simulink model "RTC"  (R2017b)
settings: Solver=FixedStepDiscrete  StartTime=0.0  StopTime=10.0  FixedStep=0.01  RelTol=1e-3  EnableMultiTasking=on
undefined symbols (not defined in the file): ASWTYPE_FALSE, ASWTYPE_TRUE, Enum_CTCCtrCtlState, Enum_ISPEcuOffTiSt, RTC_CONST0_NUMB, RTC_CONST1000_NUMB, RTC_CONST4294967000_NUMB, RTC_CONST60_NUMB, RTC_CONST86400_NUMB, RTC_RUNTIME_MS
libraries: AIWAYS_Powertrain_BMS_lib x32

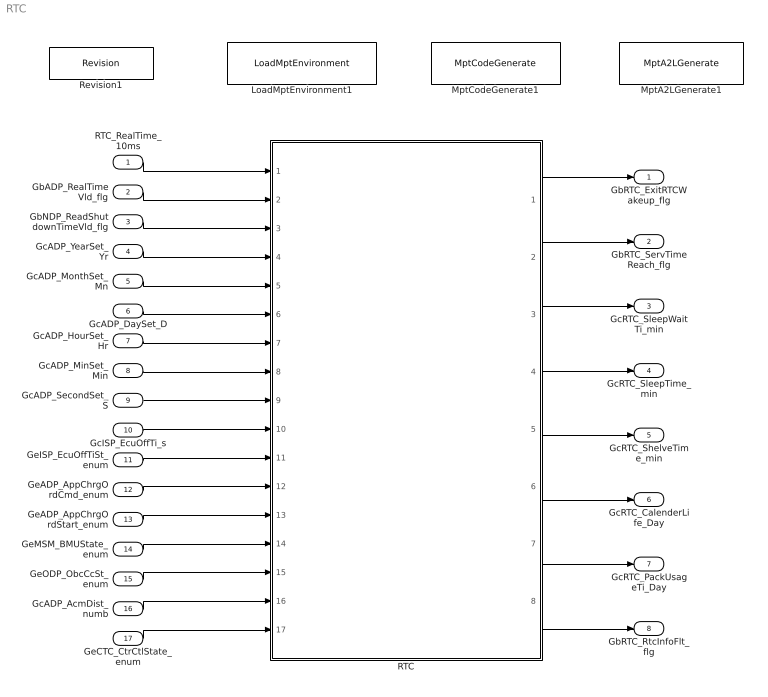
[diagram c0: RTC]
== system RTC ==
  RTC_RealTime_10ms : Inport
  GbADP_RealTimeVld_flg : Inport  Port=2
  GbNDP_ReadShutdownTimeVld_flg : Inport  Port=3
  GcADP_YearSet_Yr : Inport  Port=4
  GcADP_MonthSet_Mn : Inport  Port=5
  GcADP_DaySet_D : Inport  Port=6
  GcADP_HourSet_Hr : Inport  Port=7
  GcADP_MinSet_Min : Inport  Port=8
  GcADP_SecondSet_S : Inport  Port=9
  GcISP_EcuOffTi_s : Inport  Port=10
  GeISP_EcuOffTiSt_enum : Inport  Port=11
  GeADP_AppChrgOrdCmd_enum : Inport  Port=12
  GeADP_AppChrgOrdStart_enum : Inport  Port=13
  GeMSM_BMUState_enum : Inport  Port=14
  GeODP_ObcCcSt_enum : Inport  Port=15
  GcADP_AcmDist_numb : Inport  Port=16
  GeCTC_CtrCtlState_enum : Inport  Port=17
  LoadMptEnvironment1 : AIWAYS_Powertrain_BMS_lib/Config/LoadMptEnvironment  ProjectName=Comm  SuppierID=NewPlatformUAES
  MptA2LGenerate1 : AIWAYS_Powertrain_BMS_lib/Config/MptA2LGenerate  SystemSampleTime=-1
  MptCodeGenerate1 : AIWAYS_Powertrain_BMS_lib/Config/MptCodeGenerate  SystemSampleTime=-1
  RTC : Subsystem
  Revision1 : AIWAYS_Powertrain_BMS_lib/Config/Revision  curVersion='M102C100'  newVersion='M102C100'
  GbRTC_ExitRTCWakeup_flg : Outport
  GbRTC_ServTimeReach_flg : Outport  Port=2
  GcRTC_SleepWaitTi_min : Outport  Port=3
  GcRTC_SleepTime_min : Outport  Port=4
  GcRTC_ShelveTime_min : Outport  Port=5
  GcRTC_CalenderLife_Day : Outport  Port=6
  GcRTC_PackUsageTi_Day : Outport  Port=7
  GbRTC_RtcInfoFlt_flg : Outport  Port=8
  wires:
  RTC_RealTime_10ms/1 -> RTC/1(RTC_RealTime_10ms)
  GbADP_RealTimeVld_flg/1 -> RTC/2(GbADP_RealTimeVld_flg)
  GbNDP_ReadShutdownTimeVld_flg/1 -> RTC/3(GbNDP_ReadShutdownTimeVld_flg)
  GcADP_YearSet_Yr/1 -> RTC/4(GcADP_YearSet_Yr)
  GcADP_MonthSet_Mn/1 -> RTC/5(GcADP_MonthSet_Mn)
  GcADP_DaySet_D/1 -> RTC/6(GcADP_DaySet_D)
  GcADP_HourSet_Hr/1 -> RTC/7(GcADP_HourSet_Hr)
  GcADP_MinSet_Min/1 -> RTC/8(GcADP_MinSet_Min)
  GcADP_SecondSet_S/1 -> RTC/9(GcADP_SecondSet_S)
  GcISP_EcuOffTi_s/1 -> RTC/10(GcISP_EcuOffTi_s)
  GeISP_EcuOffTiSt_enum/1 -> RTC/11(GeISP_EcuOffTiSt_enum)
  GeADP_AppChrgOrdCmd_enum/1 -> RTC/12(GeADP_AppChrgOrdCmd_enum)
  GeADP_AppChrgOrdStart_enum/1 -> RTC/13(GeADP_AppChrgOrdStart_enum)
  GeMSM_BMUState_enum/1 -> RTC/14(GeMSM_BMUState_enum)
  GeODP_ObcCcSt_enum/1 -> RTC/15(GeODP_ObcCcSt_enum)
  GcADP_AcmDist_numb/1 -> RTC/16(GcADP_AcmDist_numb)
  GeCTC_CtrCtlState_enum/1 -> RTC/17(GeCTC_CtrCtlState_enum)
  RTC/1(GbRTC_ExitRTCWakeup_flg) -> GbRTC_ExitRTCWakeup_flg/1
  RTC/2(GbRTC_ServTimeReach_flg) -> GbRTC_ServTimeReach_flg/1
  RTC/3(GcRTC_SleepWaitTi_min) -> GcRTC_SleepWaitTi_min/1
  RTC/4(GcRTC_SleepTime_min) -> GcRTC_SleepTime_min/1
  RTC/5(GcRTC_ShelveTime_min) -> GcRTC_ShelveTime_min/1
  RTC/6(GcRTC_CalenderLife_Day) -> GcRTC_CalenderLife_Day/1
  RTC/7(GcRTC_PackUsageTi_Day) -> GcRTC_PackUsageTi_Day/1
  RTC/8(GbRTC_RtcInfoFlt_flg) -> GbRTC_RtcInfoFlt_flg/1

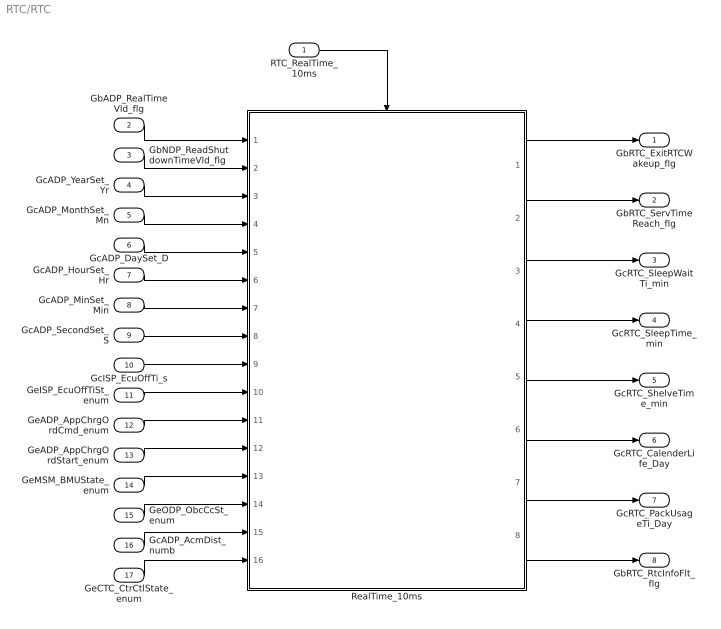
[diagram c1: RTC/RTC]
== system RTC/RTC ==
  RTC_RealTime_10ms : Inport
  GbADP_RealTimeVld_flg : Inport  Port=2
  GbNDP_ReadShutdownTimeVld_flg : Inport  Port=3
  GcADP_YearSet_Yr : Inport  Port=4
  GcADP_MonthSet_Mn : Inport  Port=5
  GcADP_DaySet_D : Inport  Port=6
  GcADP_HourSet_Hr : Inport  Port=7
  GcADP_MinSet_Min : Inport  Port=8
  GcADP_SecondSet_S : Inport  Port=9
  GcISP_EcuOffTi_s : Inport  Port=10
  GeISP_EcuOffTiSt_enum : Inport  Port=11
  GeADP_AppChrgOrdCmd_enum : Inport  Port=12
  GeADP_AppChrgOrdStart_enum : Inport  Port=13
  GeMSM_BMUState_enum : Inport  Port=14
  GeODP_ObcCcSt_enum : Inport  Port=15
  GcADP_AcmDist_numb : Inport  Port=16
  GeCTC_CtrCtlState_enum : Inport  Port=17
  RealTime_10ms : Subsystem
  GbRTC_ExitRTCWakeup_flg : Outport
  GbRTC_ServTimeReach_flg : Outport  Port=2
  GcRTC_SleepWaitTi_min : Outport  Port=3
  GcRTC_SleepTime_min : Outport  Port=4
  GcRTC_ShelveTime_min : Outport  Port=5
  GcRTC_CalenderLife_Day : Outport  Port=6
  GcRTC_PackUsageTi_Day : Outport  Port=7
  GbRTC_RtcInfoFlt_flg : Outport  Port=8
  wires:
  RTC_RealTime_10ms/1 -> RealTime_10ms/Trigger
  GbADP_RealTimeVld_flg/1 -> RealTime_10ms/1(GbADP_RealTimeVld_flg)
  GbNDP_ReadShutdownTimeVld_flg/1 -> RealTime_10ms/2(GbNDP_ReadShutdownTimeVld_flg)
  GcADP_YearSet_Yr/1 -> RealTime_10ms/3(GcADP_YearSet_Yr)
  GcADP_MonthSet_Mn/1 -> RealTime_10ms/4(GcADP_MonthSet_Mn)
  GcADP_DaySet_D/1 -> RealTime_10ms/5(GcADP_DaySet_D)
  GcADP_HourSet_Hr/1 -> RealTime_10ms/6(GcADP_HourSet_Hr)
  GcADP_MinSet_Min/1 -> RealTime_10ms/7(GcADP_MinSet_Min)
  GcADP_SecondSet_S/1 -> RealTime_10ms/8(GcADP_SecondSet_S)
  GcISP_EcuOffTi_s/1 -> RealTime_10ms/9(GcISP_EcuOffTi_s)
  GeISP_EcuOffTiSt_enum/1 -> RealTime_10ms/10(GeISP_EcuOffTiSt_enum)
  GeADP_AppChrgOrdCmd_enum/1 -> RealTime_10ms/11(GeADP_AppChrgOrdCmd_enum)
  GeADP_AppChrgOrdStart_enum/1 -> RealTime_10ms/12(GeADP_AppChrgOrdStart_enum)
  GeMSM_BMUState_enum/1 -> RealTime_10ms/13(GeMSM_BMUState_enum)
  GeODP_ObcCcSt_enum/1 -> RealTime_10ms/14(GeODP_ObcCcSt_enum)
  GcADP_AcmDist_numb/1 -> RealTime_10ms/15(GcADP_AcmDist_numb)
  GeCTC_CtrCtlState_enum/1 -> RealTime_10ms/16(GeCTC_CtrCtlState_enum)
  RealTime_10ms/1(GbRTC_ExitRTCWakeup_flg) -> GbRTC_ExitRTCWakeup_flg/1
  RealTime_10ms/2(GbRTC_ServTimeReach_flg) -> GbRTC_ServTimeReach_flg/1
  RealTime_10ms/3(GcRTC_SleepWaitTi_min) -> GcRTC_SleepWaitTi_min/1
  RealTime_10ms/4(GcRTC_SleepTime_min) -> GcRTC_SleepTime_min/1
  RealTime_10ms/5(GcRTC_ShelveTime_min) -> GcRTC_ShelveTime_min/1
  RealTime_10ms/6(GcRTC_CalenderLife_Day) -> GcRTC_CalenderLife_Day/1
  RealTime_10ms/7(GcRTC_PackUsageTi_Day) -> GcRTC_PackUsageTi_Day/1
  RealTime_10ms/8(GbRTC_RtcInfoFlt_flg) -> GbRTC_RtcInfoFlt_flg/1

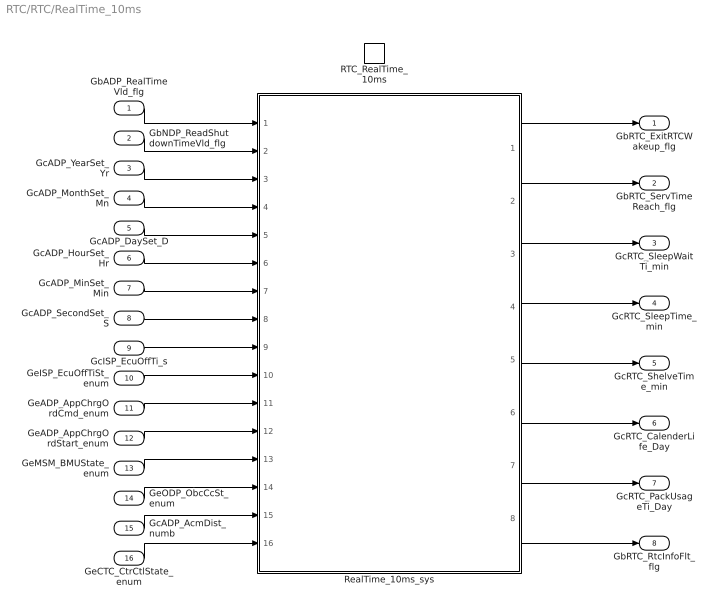
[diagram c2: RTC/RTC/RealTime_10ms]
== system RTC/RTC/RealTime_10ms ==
  GbADP_RealTimeVld_flg : Inport
  GbNDP_ReadShutdownTimeVld_flg : Inport  Port=2
  GcADP_YearSet_Yr : Inport  Port=3
  GcADP_MonthSet_Mn : Inport  Port=4
  GcADP_DaySet_D : Inport  Port=5
  GcADP_HourSet_Hr : Inport  Port=6
  GcADP_MinSet_Min : Inport  Port=7
  GcADP_SecondSet_S : Inport  Port=8
  GcISP_EcuOffTi_s : Inport  Port=9
  GeISP_EcuOffTiSt_enum : Inport  Port=10
  GeADP_AppChrgOrdCmd_enum : Inport  Port=11
  GeADP_AppChrgOrdStart_enum : Inport  Port=12
  GeMSM_BMUState_enum : Inport  Port=13
  GeODP_ObcCcSt_enum : Inport  Port=14
  GcADP_AcmDist_numb : Inport  Port=15
  GeCTC_CtrCtlState_enum : Inport  Port=16
  RTC_RealTime_10ms : TriggerPort  TriggerType=function-call  VariantControl=(inherit)
  RealTime_10ms_sys : Subsystem
  GbRTC_ExitRTCWakeup_flg : Outport
  GbRTC_ServTimeReach_flg : Outport  Port=2
  GcRTC_SleepWaitTi_min : Outport  Port=3
  GcRTC_SleepTime_min : Outport  Port=4
  GcRTC_ShelveTime_min : Outport  Port=5
  GcRTC_CalenderLife_Day : Outport  Port=6
  GcRTC_PackUsageTi_Day : Outport  Port=7
  GbRTC_RtcInfoFlt_flg : Outport  Port=8
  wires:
  GbADP_RealTimeVld_flg/1 -> RealTime_10ms_sys/1(GbADP_RealTimeVld_flg)
  GbNDP_ReadShutdownTimeVld_flg/1 -> RealTime_10ms_sys/2(GbNDP_ReadShutdownTimeVld_flg)
  GcADP_YearSet_Yr/1 -> RealTime_10ms_sys/3(GcADP_YearSet_Yr)
  GcADP_MonthSet_Mn/1 -> RealTime_10ms_sys/4(GcADP_MonthSet_Mn)
  GcADP_DaySet_D/1 -> RealTime_10ms_sys/5(GcADP_DaySet_D)
  GcADP_HourSet_Hr/1 -> RealTime_10ms_sys/6(GcADP_HourSet_Hr)
  GcADP_MinSet_Min/1 -> RealTime_10ms_sys/7(GcADP_MinSet_Min)
  GcADP_SecondSet_S/1 -> RealTime_10ms_sys/8(GcADP_SecondSet_S)
  GcISP_EcuOffTi_s/1 -> RealTime_10ms_sys/9(GcISP_EcuOffTi_s)
  GeISP_EcuOffTiSt_enum/1 -> RealTime_10ms_sys/10(GeISP_EcuOffTiSt_enum)
  GeADP_AppChrgOrdCmd_enum/1 -> RealTime_10ms_sys/11(GeADP_AppChrgOrdCmd_enum)
  GeADP_AppChrgOrdStart_enum/1 -> RealTime_10ms_sys/12(GeADP_AppChrgOrdStart_enum)
  GeMSM_BMUState_enum/1 -> RealTime_10ms_sys/13(GeMSM_BMUState_enum)
  GeODP_ObcCcSt_enum/1 -> RealTime_10ms_sys/14(GeODP_ObcCcSt_enum)
  GcADP_AcmDist_numb/1 -> RealTime_10ms_sys/15(GcADP_AcmDist_numb)
  GeCTC_CtrCtlState_enum/1 -> RealTime_10ms_sys/16(GeCTC_CtrCtlState_enum)
  RealTime_10ms_sys/1(GbRTC_ExitRTCWakeup_flg) -> GbRTC_ExitRTCWakeup_flg/1
  RealTime_10ms_sys/2(GbRTC_ServTimeReach_flg) -> GbRTC_ServTimeReach_flg/1
  RealTime_10ms_sys/3(GcRTC_SleepWaitTi_min) -> GcRTC_SleepWaitTi_min/1
  RealTime_10ms_sys/4(GcRTC_SleepTime_min) -> GcRTC_SleepTime_min/1
  RealTime_10ms_sys/5(GcRTC_ShelveTime_min) -> GcRTC_ShelveTime_min/1
  RealTime_10ms_sys/6(GcRTC_CalenderLife_Day) -> GcRTC_CalenderLife_Day/1
  RealTime_10ms_sys/7(GcRTC_PackUsageTi_Day) -> GcRTC_PackUsageTi_Day/1
  RealTime_10ms_sys/8(GbRTC_RtcInfoFlt_flg) -> GbRTC_RtcInfoFlt_flg/1

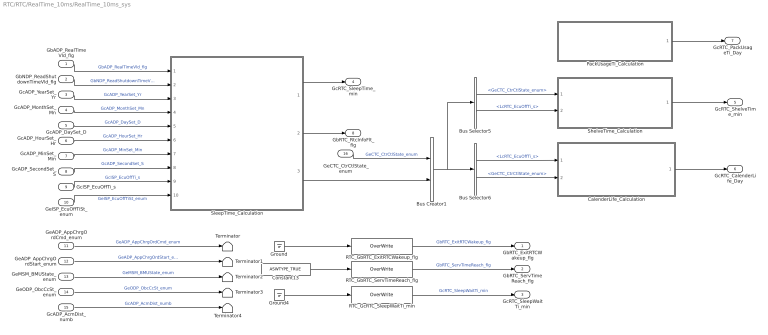
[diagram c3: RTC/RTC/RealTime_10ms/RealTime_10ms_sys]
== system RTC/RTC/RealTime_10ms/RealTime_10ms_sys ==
  GbADP_RealTimeVld_flg : Inport
  GbNDP_ReadShutdownTimeVld_flg : Inport  Port=2
  GcADP_YearSet_Yr : Inport  Port=3
  GcADP_MonthSet_Mn : Inport  Port=4
  GcADP_DaySet_D : Inport  Port=5
  GcADP_HourSet_Hr : Inport  Port=6
  GcADP_MinSet_Min : Inport  Port=7
  GcADP_SecondSet_S : Inport  Port=8
  GcISP_EcuOffTi_s : Inport  Port=9
  GeISP_EcuOffTiSt_enum : Inport  Port=10
  GeADP_AppChrgOrdCmd_enum : Inport  Port=11
  GeADP_AppChrgOrdStart_enum : Inport  Port=12
  GeMSM_BMUState_enum : Inport  Port=13
  GeODP_ObcCcSt_enum : Inport  Port=14
  GcADP_AcmDist_numb : Inport  Port=15
  GeCTC_CtrCtlState_enum : Inport  Port=16
  Bus Creator1 : BusCreator  Inputs=2
  Bus Selector5 : BusSelector  OutputSignals=GeCTC_CtrCtlState_enum,LcRTC_EcuOffTi_s
  Bus Selector6 : BusSelector  OutputSignals=LcRTC_EcuOffTi_s,GeCTC_CtrCtlState_enum
  CalenderLife_Calculation : Subsystem
  Constant13 : Constant  Value=ASWTYPE_TRUE
  Ground : Ground
  Ground4 : Ground
  PackUsageTi_Calculation : Subsystem
  RTC_GbRTC_ExitRTCWakeup_flg : AIWAYS_Powertrain_BMS_lib/Signals/OverWrite  OverWrite_Value=CbRTC_ExitRTCWakeupOvr_flg  OverWrite_flag=CbRTC_ExitRTCWakeupOvrSwt_flg
  RTC_GbRTC_ServTimeReach_flg : AIWAYS_Powertrain_BMS_lib/Signals/OverWrite  OverWrite_Value=CbRTC_ServTimeReachOvr_flg  OverWrite_flag=CbRTC_ServTimeReachOvrSwt_flg
  RTC_GcRTC_SleepWaitTi_min : AIWAYS_Powertrain_BMS_lib/Signals/OverWrite  OverWrite_Value=CcRTC_SleepWaitTiOvr_min  OverWrite_flag=CbRTC_SleepWaitTiOvrSwt_flg
  ShelveTime_Calculation : Subsystem
  SleepTime_Calculation : Subsystem
  Terminator{,1..4} (5 alike) : Terminator
  GbRTC_ExitRTCWakeup_flg : Outport
  GbRTC_ServTimeReach_flg : Outport  Port=2
  GcRTC_SleepWaitTi_min : Outport  Port=3
  GcRTC_SleepTime_min : Outport  Port=4
  GcRTC_ShelveTime_min : Outport  Port=5
  GcRTC_CalenderLife_Day : Outport  Port=6
  GcRTC_PackUsageTi_Day : Outport  Port=7
  GbRTC_RtcInfoFlt_flg : Outport  Port=8
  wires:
  GeADP_AppChrgOrdCmd_enum/1 -> Terminator/1  "GeADP_AppChrgOrdCmd_enum"
  GeADP_AppChrgOrdStart_enum/1 -> Terminator1/1  "GeADP_AppChrgOrdStart_enum"
  GeODP_ObcCcSt_enum/1 -> Terminator3/1  "GeODP_ObcCcSt_enum"
  GeMSM_BMUState_enum/1 -> Terminator2/1  "GeMSM_BMUState_enum"
  RTC_GbRTC_ExitRTCWakeup_flg/1 -> GbRTC_ExitRTCWakeup_flg/1  "GbRTC_ExitRTCWakeup_flg"
  RTC_GbRTC_ServTimeReach_flg/1 -> GbRTC_ServTimeReach_flg/1  "GbRTC_ServTimeReach_flg"
  RTC_GcRTC_SleepWaitTi_min/1 -> GcRTC_SleepWaitTi_min/1  "GcRTC_SleepWaitTi_min"
  Ground/1 -> RTC_GbRTC_ExitRTCWakeup_flg/1
  Constant13/1 -> RTC_GbRTC_ServTimeReach_flg/1
  Ground4/1 -> RTC_GcRTC_SleepWaitTi_min/1
  SleepTime_Calculation/1(GcRTC_SleepTime_min) -> GcRTC_SleepTime_min/1
  ShelveTime_Calculation/1(GcRTC_ShelveTime_min) -> GcRTC_ShelveTime_min/1
  PackUsageTi_Calculation/1(GcRTC_PackUsageTi_Day) -> GcRTC_PackUsageTi_Day/1
  GcADP_AcmDist_numb/1 -> Terminator4/1  "GcADP_AcmDist_numb"
  GbADP_RealTimeVld_flg/1 -> SleepTime_Calculation/1(GbADP_RealTimeVld_flg)  "GbADP_RealTimeVld_flg"
  GbNDP_ReadShutdownTimeVld_flg/1 -> SleepTime_Calculation/2(GbNDP_ReadShutdownTimeVld_flg)  "GbNDP_ReadShutdownTimeVld_flg"
  GcADP_YearSet_Yr/1 -> SleepTime_Calculation/3(GcADP_YearSet_Yr)  "GcADP_YearSet_Yr"
  GcADP_MonthSet_Mn/1 -> SleepTime_Calculation/4(GcADP_MonthSet_Mn)  "GcADP_MonthSet_Mn"
  GcADP_DaySet_D/1 -> SleepTime_Calculation/5(GcADP_DaySet_D)  "GcADP_DaySet_D"
  GcADP_HourSet_Hr/1 -> SleepTime_Calculation/6(GcADP_HourSet_Hr)  "GcADP_HourSet_Hr"
  GcADP_MinSet_Min/1 -> SleepTime_Calculation/7(GcADP_MinSet_Min)  "GcADP_MinSet_Min"
  GcADP_SecondSet_S/1 -> SleepTime_Calculation/8(GcADP_SecondSet_S)  "GcADP_SecondSet_S"
  GeISP_EcuOffTiSt_enum/1 -> SleepTime_Calculation/10(GeISP_EcuOffTiSt_enum)  "GeISP_EcuOffTiSt_enum"
  GcISP_EcuOffTi_s/1 -> SleepTime_Calculation/9(GcISP_EcuOffTi_s)  "GcISP_EcuOffTi_s"
  GeCTC_CtrCtlState_enum/1 -> Bus Creator1/1  "GeCTC_CtrCtlState_enum"
  SleepTime_Calculation/3(LcRTC_EcuOffTi_s) -> Bus Creator1/2
  Bus Creator1/1 -> Bus Selector6/1, Bus Selector5/1
  Bus Selector5/1 -> ShelveTime_Calculation/1(GeCTC_CtrCtlState_enum)  "<GeCTC_CtrCtlState_enum>"
  Bus Selector5/2 -> ShelveTime_Calculation/2(LcRTC_EcuOffTi_s)  "<LcRTC_EcuOffTi_s>"
  CalenderLife_Calculation/1(GcRTC_CalenderLife_Day) -> GcRTC_CalenderLife_Day/1
  SleepTime_Calculation/2(GbRTC_RtcInfoFlt_flg) -> GbRTC_RtcInfoFlt_flg/1
  Bus Selector6/1 -> CalenderLife_Calculation/1(LcRTC_EcuOffTi_s)  "<LcRTC_EcuOffTi_s>"
  Bus Selector6/2 -> CalenderLife_Calculation/2(GeCTC_CtrCtlState_enum)  "<GeCTC_CtrCtlState_enum>"

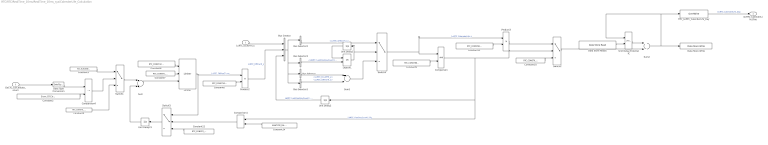
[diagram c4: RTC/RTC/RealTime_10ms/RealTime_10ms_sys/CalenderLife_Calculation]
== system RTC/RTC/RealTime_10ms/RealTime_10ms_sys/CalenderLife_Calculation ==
  LcRTC_EcuOffTi_s : Inport
  GeCTC_CtrCtlState_enum : Inport  Port=2
  Bus Creator : BusCreator  Inputs=3
  Bus Selector : BusSelector  OutputSignals=LcRTC_EcuOffTi_s
  Bus Selector1 : BusSelector  OutputSignals=LcRTC_OfflineTi_s
  Bus Selector2 : BusSelector  OutputSignals=LcRTC_OfflineTi_s
  Bus Selector3 : BusSelector  OutputSignals=LbRTC_LastOneDayCount1_flg
  Comparison : RelationalOperator  OutDataTypeStr=boolean
  Comparison1 : RelationalOperator  Operator===  OutDataTypeStr=boolean
  Comparison4 : RelationalOperator  Operator=~=  OutDataTypeStr=boolean
  Constant{4,7,10,12} (4 alike) : Constant  Value=RTC_CONST0_NUMB
  Constant11 : Constant  Value=RTC_CONST86400_NUMB
  Constant14 : Constant  Value=ASWTYPE_FALSE
  Constant2 : Constant  Value=Enum_CTCCtrCtlState.Enum_CTCCtrCtlState_Online
  Constant3 : Constant  Value=RTC_RUNTIME_MS
  Constant6 : Constant  Value=RTC_CONST1000_NUMB
  Constant8 : Constant  Value=RTC_CONST4294967000_NUMB
  Constant9 : Constant  Value=RTC_CONST86400_NUMB
  Data Store Read1 : AIWAYS_Powertrain_BMS_lib/Signals/Data Store Read  Priority=0  DSR=EcNVM_CalenderLife_Day
  Data Store Write : AIWAYS_Powertrain_BMS_lib/Signals/Data Store Write  DSW=EcNVM_CalenderLife_Day
  Data Type Conversion : DataTypeConversion
  Limiter : AIWAYS_Powertrain_BMS_lib/Nonlinear Blocks/Limiter
  Logical1 : Logic  Operator=OR  OutDataTypeStr=boolean
  Product2 : Product  Inputs=*/  OutDataTypeStr=Inherit: Inherit via back propagation
  Product3 : Product  Inputs=*/  OutDataTypeStr=uint32  RndMeth=Round
  RTC_GcRTC_CalenderLife_Day : AIWAYS_Powertrain_BMS_lib/Signals/OverWrite  OverWrite_Value=CcRTC_CalenderLifeOvr_Day  OverWrite_flag=CbRTC_CalenderLifeOvrSwt_flg
  Sum : Sum  OutDataTypeStr=uint32  RndMeth=Zero
  Sum1 : Sum  OutDataTypeStr=Inherit: Inherit via back propagation  RndMeth=Zero
  Sum2 : Sum  OutDataTypeStr=Inherit: Inherit via back propagation  RndMeth=Zero
  Switch{1..4} (4 alike) : Switch  Criteria=u2 ~= 0  Threshold=1  RndMeth=Zero
  Unit Delay External IC : AIWAYS_Powertrain_BMS_lib/Delay Blocks/Unit Delay External IC
  Unit Delay1 : UnitDelay  InitialCondition=ASWTYPE_FALSE  SampleTime=-1  StateName=StateName
  Unit Delay2 : UnitDelay  InitialCondition=ASWTYPE_FALSE  SampleTime=-1  StateName=StateName
  Unit Delay21 : UnitDelay  SampleTime=-1  StateName=StateName
  GcRTC_CalenderLife_Day : Outport
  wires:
  Comparison4/1 -> Switch1/2
  Switch1/1 -> Sum/1
  Switch2/1 -> Sum2/2
  Sum1/1 -> Switch4/3
  Constant6/1 -> Product2/2
  Switch4/1 -> Product3/1, Comparison/1  "LcRTC_CalenderLife_s"
  Product3/1 -> Switch2/1
  Bus Selector2/1 -> Switch4/1  "<LcRTC_OfflineTi_s>"
  Constant14/1 -> Comparison1/2
  Constant10/1 -> Switch2/3
  Constant7/1 -> Limiter/2
  Constant8/1 -> Limiter/1
  Logical1/1 -> Unit Delay1/1, Switch4/2
  Unit Delay1/1 -> Logical1/1
  Data Type Conversion/1 -> Comparison4/1
  Constant2/1 -> Comparison4/2
  Bus Creator/1 -> Bus Selector1/1, Bus Selector/1, Bus Selector3/1, Bus Selector2/1
  Limiter/1 -> Switch3/1, Product2/1  "LcRTC_OfflineTi_ms"
  Bus Selector/1 -> Sum1/1  "<LcRTC_EcuOffTi_s>"
  Product2/1 -> Bus Creator/2  "LcRTC_OfflineTi_s"
  Bus Selector3/1 -> Logical1/2  "<LbRTC_LastOneDayCount1_flg>"
  Constant11/1 -> Product3/2
  Bus Selector1/1 -> Sum1/2  "<LcRTC_OfflineTi_s>"
  LcRTC_EcuOffTi_s/1 -> Bus Creator/1
  Unit Delay2/1 -> Bus Creator/3  "LbRTC_LastOneDayCount1_flg"
  GeCTC_CtrCtlState_enum/1 -> Data Type Conversion/1
  Data Store Read1/1 -> Unit Delay External IC/2
  Switch3/1 -> Unit Delay21/1
  Constant12/1 -> Switch3/3
  Comparison/1 -> Comparison1/1, Unit Delay2/1, Switch2/2  "LbRTC_OneDayCount1_flg"
  Constant9/1 -> Comparison/2
  Unit Delay External IC/1 -> Sum2/1
  Unit Delay21/1 -> Sum/2
  Sum/1 -> Limiter/3
  Constant4/1 -> Switch1/3
  Constant3/1 -> Switch1/1
  Comparison1/1 -> Switch3/2
  RTC_GcRTC_CalenderLife_Day/1 -> GcRTC_CalenderLife_Day/1  "GcRTC_CalenderLife_Day"
  Sum2/1 -> Data Store Write/1, RTC_GcRTC_CalenderLife_Day/1, Unit Delay External IC/1

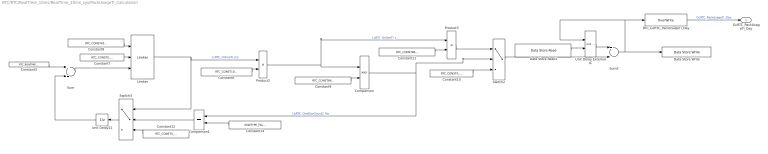
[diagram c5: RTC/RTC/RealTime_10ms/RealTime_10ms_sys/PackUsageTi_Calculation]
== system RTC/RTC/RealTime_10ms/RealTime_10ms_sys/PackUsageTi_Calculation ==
  Comparison : RelationalOperator  OutDataTypeStr=boolean
  Comparison1 : RelationalOperator  Operator===  OutDataTypeStr=boolean
  Constant10 : Constant  Value=RTC_CONST0_NUMB
  Constant11 : Constant  Value=RTC_CONST86400_NUMB
  Constant12 : Constant  Value=RTC_CONST0_NUMB
  Constant14 : Constant  Value=ASWTYPE_FALSE
  Constant3 : Constant  Value=RTC_RUNTIME_MS
  Constant6 : Constant  Value=RTC_CONST1000_NUMB
  Constant7 : Constant  Value=RTC_CONST0_NUMB
  Constant8 : Constant  Value=RTC_CONST4294967000_NUMB
  Constant9 : Constant  Value=RTC_CONST86400_NUMB
  Data Store Read1 : AIWAYS_Powertrain_BMS_lib/Signals/Data Store Read  Priority=0  DSR=EcNVM_PackUsageTi_Day
  Data Store Write : AIWAYS_Powertrain_BMS_lib/Signals/Data Store Write  DSW=EcNVM_PackUsageTi_Day
  Limiter : AIWAYS_Powertrain_BMS_lib/Nonlinear Blocks/Limiter
  Product2 : Product  Inputs=*/  OutDataTypeStr=Inherit: Inherit via back propagation
  Product3 : Product  Inputs=*/  OutDataTypeStr=uint32  RndMeth=Round
  RTC_GcRTC_PackUsageTi_Day : AIWAYS_Powertrain_BMS_lib/Signals/OverWrite  OverWrite_Value=CcRTC_PackUsageTiOvr_Day  OverWrite_flag=CbRTC_PackUsageTiOvrSwt_flg
  Sum : Sum  OutDataTypeStr=uint32  RndMeth=Zero
  Sum2 : Sum  OutDataTypeStr=Inherit: Inherit via back propagation  RndMeth=Zero
  Switch2 : Switch  Criteria=u2 ~= 0  Threshold=1  RndMeth=Zero
  Switch3 : Switch  Criteria=u2 ~= 0  Threshold=1  RndMeth=Zero
  Unit Delay External IC : AIWAYS_Powertrain_BMS_lib/Delay Blocks/Unit Delay External IC
  Unit Delay21 : UnitDelay  SampleTime=-1  StateName=StateName
  GcRTC_PackUsageTi_Day : Outport
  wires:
  Comparison1/1 -> Switch3/2
  Sum/1 -> Limiter/3
  Unit Delay21/1 -> Sum/2
  Unit Delay External IC/1 -> Sum2/1
  Constant9/1 -> Comparison/2
  Comparison/1 -> Switch2/2, Comparison1/1  "LbRTC_OneDayCount2_flg"
  Constant12/1 -> Switch3/3
  Switch3/1 -> Unit Delay21/1
  Data Store Read1/1 -> Unit Delay External IC/2
  Constant11/1 -> Product3/2
  Product2/1 -> Comparison/1, Product3/1  "LcRTC_OnlineTi_s"
  Limiter/1 -> Product2/1, Switch3/1  "LcRTC_OnlineTi_ms"
  Constant8/1 -> Limiter/1
  Constant7/1 -> Limiter/2
  Constant10/1 -> Switch2/3
  Constant14/1 -> Comparison1/2
  Product3/1 -> Switch2/1
  Constant6/1 -> Product2/2
  Switch2/1 -> Sum2/2
  Constant3/1 -> Sum/1
  RTC_GcRTC_PackUsageTi_Day/1 -> GcRTC_PackUsageTi_Day/1  "GcRTC_PackUsageTi_Day"
  Sum2/1 -> Unit Delay External IC/1, RTC_GcRTC_PackUsageTi_Day/1, Data Store Write/1

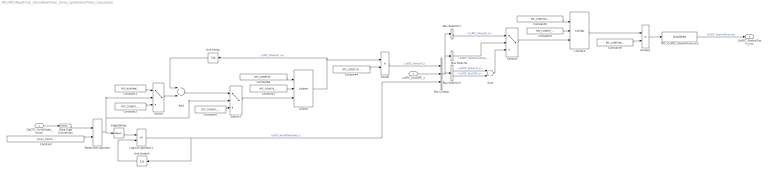
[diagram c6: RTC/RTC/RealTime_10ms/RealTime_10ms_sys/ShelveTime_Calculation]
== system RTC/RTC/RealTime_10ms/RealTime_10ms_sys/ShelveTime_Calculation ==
  GeCTC_CtrCtlState_enum : Inport
  LcRTC_EcuOffTi_s : Inport  Port=2
  Add : Sum  OutDataTypeStr=uint32
  Bus Creator : BusCreator  Inputs=3
  Bus Selector : BusSelector  OutputSignals=LbRTC_NotOfflineState_flg
  Bus Selector1 : BusSelector  OutputSignals=LcRTC_ShelveTi_s
  Bus Selector2 : BusSelector  OutputSignals=LcRTC_ShelveTi_s,LcRTC_EcuOffTi_s
  Constant : Constant  Value=Enum_CTCCtrCtlState.Enum_CTCCtrCtlState_Offline
  Constant1 : Constant  Value=RTC_RUNTIME_MS
  Constant{2..3,5,7} (4 alike) : Constant  Value=RTC_CONST0_NUMB
  Constant4 : Constant  Value=RTC_CONST1000_NUMB
  Constant6 : Constant  Value=RTC_CONST4294967000_NUMB
  Constant8 : Constant  Value=RTC_CONST4294967000_NUMB
  Constant9 : Constant  Value=RTC_CONST60_NUMB
  Data Type Conversion : DataTypeConversion
  Divide : Product  Inputs=*/  OutDataTypeStr=uint32
  Divide1 : Product  Inputs=*/  OutDataTypeStr=uint32
  EdgeFalling : AIWAYS_Powertrain_BMS_lib/Logical Operators/EdgeFalling
  Limiter : AIWAYS_Powertrain_BMS_lib/Nonlinear Blocks/Limiter
  Limiter1 : AIWAYS_Powertrain_BMS_lib/Nonlinear Blocks/Limiter
  Logical Operator1 : Logic  Operator=OR  AllPortsSameDT=off  OutDataTypeStr=boolean
  RTC_GcRTC_ShelveTime_min : AIWAYS_Powertrain_BMS_lib/Signals/OverWrite  OverWrite_Value=CcRTC_ShelveTimeOvr_min  OverWrite_flag=CbRTC_ShelveTimeOvrSwt_flg
  Relational Operator : RelationalOperator  Operator===  OutDataTypeStr=boolean
  Sum : Sum  OutDataTypeStr=Inherit: Inherit via back propagation  RndMeth=Zero
  Switch : Switch  Criteria=u2 ~= 0
  Switch2 : Switch  Criteria=u2 ~= 0
  Switch3 : Switch  Criteria=u2 ~= 0  OutDataTypeStr=uint32
  Unit Delay : UnitDelay  SampleTime=-1  StateName=StateName
  Unit Delay2 : UnitDelay  SampleTime=-1  StateName=StateName
  GcRTC_ShelveTime_min : Outport
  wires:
  RTC_GcRTC_ShelveTime_min/1 -> GcRTC_ShelveTime_min/1  "GcRTC_ShelveTime_min"
  LcRTC_EcuOffTi_s/1 -> Bus Creator/2
  Unit Delay2/1 -> Logical Operator1/2
  Data Type Conversion/1 -> Relational Operator/1
  Constant/1 -> Relational Operator/2
  Constant2/1 -> Switch/3
  Constant1/1 -> Switch/1
  Logical Operator1/1 -> Bus Creator/3, Unit Delay2/1  "LbRTC_NotOfflineState_flg"
  Divide/1 -> Bus Creator/1  "LcRTC_ShelveTi_s"
  GeCTC_CtrCtlState_enum/1 -> Data Type Conversion/1
  Constant8/1 -> Limiter/1
  Constant7/1 -> Limiter/2
  EdgeFalling/1 -> Logical Operator1/1
  Constant4/1 -> Divide/2
  Relational Operator/1 -> Switch3/2, Switch/2, EdgeFalling/1
  Unit Delay/1 -> Add/1
  Switch/1 -> Add/2
  Add/1 -> Switch3/1
  Constant5/1 -> Switch3/3
  Switch3/1 -> Limiter/3
  Limiter/1 -> Divide/1, Unit Delay/1  "LcRTC_ShelveTi_ms"
  Bus Creator/1 -> Bus Selector1/1, Bus Selector/1, Bus Selector2/1
  Bus Selector/1 -> Switch2/2  "<LbRTC_NotOfflineState_flg>"
  Bus Selector1/1 -> Switch2/1  "<LcRTC_ShelveTi_s>"
  Bus Selector2/1 -> Sum/1  "<LcRTC_ShelveTi_s>"
  Bus Selector2/2 -> Sum/2  "<LcRTC_EcuOffTi_s>"
  Sum/1 -> Switch2/3
  Switch2/1 -> Limiter1/3
  Constant3/1 -> Limiter1/2
  Constant6/1 -> Limiter1/1
  Limiter1/1 -> Divide1/1
  Constant9/1 -> Divide1/2
  Divide1/1 -> RTC_GcRTC_ShelveTime_min/1

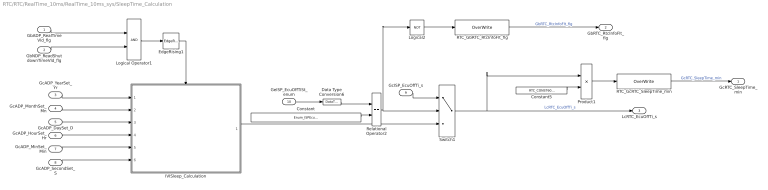
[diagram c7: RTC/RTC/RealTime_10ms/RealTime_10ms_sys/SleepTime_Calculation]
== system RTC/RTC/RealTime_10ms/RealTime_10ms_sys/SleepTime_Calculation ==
  GbADP_RealTimeVld_flg : Inport
  GbNDP_ReadShutdownTimeVld_flg : Inport  Port=2
  GcADP_YearSet_Yr : Inport  Port=3
  GcADP_MonthSet_Mn : Inport  Port=4
  GcADP_DaySet_D : Inport  Port=5
  GcADP_HourSet_Hr : Inport  Port=6
  GcADP_MinSet_Min : Inport  Port=7
  GcADP_SecondSet_S : Inport  Port=8
  GcISP_EcuOffTi_s : Inport  Port=9
  GeISP_EcuOffTiSt_enum : Inport  Port=10
  Constant : Constant  Value=Enum_ISPEcuOffTiSt.Enum_ISPEcuOffTiSt_Valid
  Constant5 : Constant  Value=RTC_CONST60_NUMB
  Data Type Conversion6 : DataTypeConversion
  EdgeRising1 : AIWAYS_Powertrain_BMS_lib/Logical Operators/EdgeRising
  IVISleep_Calculation : Subsystem
  Logical Operator1 : Logic  AllPortsSameDT=off  OutDataTypeStr=boolean
  Logical2 : Logic  Operator=NOT  OutDataTypeStr=boolean
  Product1 : Product  Inputs=*/  OutDataTypeStr=Inherit: Inherit via back propagation
  RTC_GbRTC_RtcInfoFlt_flg : AIWAYS_Powertrain_BMS_lib/Signals/OverWrite  OverWrite_Value=CbRTC_RtcInfoFltOvr_flg  OverWrite_flag=CbRTC_RtcInfoFltOvrSwt_flg
  RTC_GcRTC_SleepTime_min : AIWAYS_Powertrain_BMS_lib/Signals/OverWrite  OverWrite_Value=CcRTC_SleepTimeOvr_min  OverWrite_flag=CbRTC_SleepTimeOvrSwt_flg
  Relational Operator2 : RelationalOperator  Operator===  OutDataTypeStr=boolean
  Switch1 : Switch  Criteria=u2 ~= 0  Threshold=1  RndMeth=Zero
  GcRTC_SleepTime_min : Outport
  GbRTC_RtcInfoFlt_flg : Outport  Port=2
  LcRTC_EcuOffTi_s : Outport  Port=3
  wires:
  GbADP_RealTimeVld_flg/1 -> Logical Operator1/1
  Logical Operator1/1 -> EdgeRising1/1
  GcADP_SecondSet_S/1 -> IVISleep_Calculation/6(GcADP_SecondSet_S)
  GbNDP_ReadShutdownTimeVld_flg/1 -> Logical Operator1/2
  GcADP_MonthSet_Mn/1 -> IVISleep_Calculation/2(GcADP_MonthSet_Mn)
  GcADP_YearSet_Yr/1 -> IVISleep_Calculation/1(GcADP_YearSet_Yr)
  GcADP_MinSet_Min/1 -> IVISleep_Calculation/5(GcADP_MinSet_Min)
  GcADP_DaySet_D/1 -> IVISleep_Calculation/3(GcADP_DaySet_D)
  GcADP_HourSet_Hr/1 -> IVISleep_Calculation/4(GcADP_HourSet_Hr)
  Data Type Conversion6/1 -> Relational Operator2/1
  GcISP_EcuOffTi_s/1 -> Switch1/1
  Constant5/1 -> Product1/2
  Switch1/1 -> LcRTC_EcuOffTi_s/1, Product1/1  "LcRTC_EcuOffTi_s"
  Constant/1 -> Relational Operator2/2
  GeISP_EcuOffTiSt_enum/1 -> Data Type Conversion6/1
  RTC_GcRTC_SleepTime_min/1 -> GcRTC_SleepTime_min/1  "GcRTC_SleepTime_min"
  Product1/1 -> RTC_GcRTC_SleepTime_min/1
  IVISleep_Calculation/1(LcRTC_IVICalSleepTime_s) -> Switch1/3
  RTC_GbRTC_RtcInfoFlt_flg/1 -> GbRTC_RtcInfoFlt_flg/1  "GbRTC_RtcInfoFlt_flg"
  Relational Operator2/1 -> Logical2/1, Switch1/2
  Logical2/1 -> RTC_GbRTC_RtcInfoFlt_flg/1
  EdgeRising1/1 -> IVISleep_Calculation/Enable

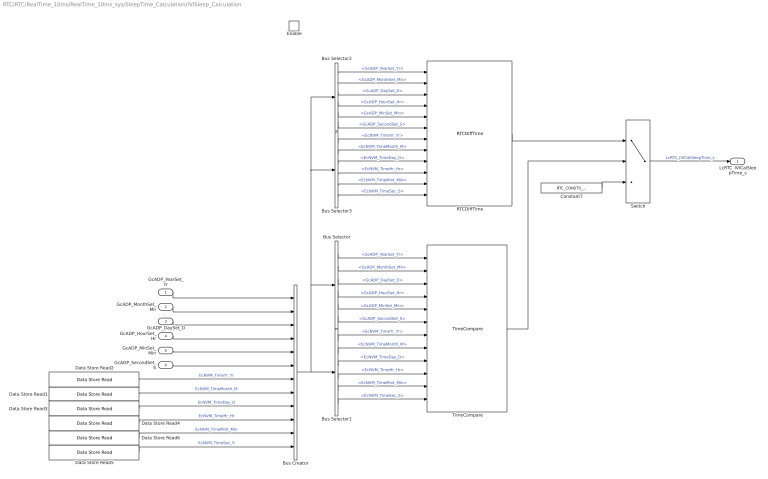
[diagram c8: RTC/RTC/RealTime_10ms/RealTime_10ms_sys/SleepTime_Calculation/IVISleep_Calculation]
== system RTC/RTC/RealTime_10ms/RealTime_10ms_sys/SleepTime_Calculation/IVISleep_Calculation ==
  GcADP_YearSet_Yr : Inport
  GcADP_MonthSet_Mn : Inport  Port=2
  GcADP_DaySet_D : Inport  Port=3
  GcADP_HourSet_Hr : Inport  Port=4
  GcADP_MinSet_Min : Inport  Port=5
  GcADP_SecondSet_S : Inport  Port=6
  Enable : EnablePort  StatesWhenEnabling=reset
  Bus Creator : BusCreator  Inputs=12
  Bus Selector : BusSelector  OutputSignals=GcADP_YearSet_Yr,GcADP_MonthSet_Mn,GcADP_DaySet_D,GcADP_HourSet_Hr,GcADP_MinSet_Min,GcADP_SecondSet_S
  Bus Selector1 : BusSelector  OutputSignals=EcNVM_TimeYr_Yr,EcNVM_TimeMonth_M,EcNVM_TimeDay_D,EcNVM_TimeHr_Hr,EcNVM_TimeMint_Min,EcNVM_TimeSec_S
  Bus Selector2 : BusSelector  OutputSignals=GcADP_YearSet_Yr,GcADP_MonthSet_Mn,GcADP_DaySet_D,GcADP_HourSet_Hr,GcADP_MinSet_Min,GcADP_SecondSet_S
  Bus Selector3 : BusSelector  OutputSignals=EcNVM_TimeYr_Yr,EcNVM_TimeMonth_M,EcNVM_TimeDay_D,EcNVM_TimeHr_Hr,EcNVM_TimeMint_Min,EcNVM_TimeSec_S
  Constant7 : Constant  Value=RTC_CONST0_NUMB
  Data Store Read1 : AIWAYS_Powertrain_BMS_lib/Signals/Data Store Read  Priority=0  DSR=EcNVM_TimeMonth_M
  Data Store Read2 : AIWAYS_Powertrain_BMS_lib/Signals/Data Store Read  Priority=0  DSR=EcNVM_TimeYr_Yr
  Data Store Read3 : AIWAYS_Powertrain_BMS_lib/Signals/Data Store Read  Priority=0  DSR=EcNVM_TimeDay_D
  Data Store Read4 : AIWAYS_Powertrain_BMS_lib/Signals/Data Store Read  Priority=0  DSR=EcNVM_TimeHr_Hr
  Data Store Read5 : AIWAYS_Powertrain_BMS_lib/Signals/Data Store Read  Priority=0  DSR=EcNVM_TimeSec_S
  Data Store Read6 : AIWAYS_Powertrain_BMS_lib/Signals/Data Store Read  Priority=0  DSR=EcNVM_TimeMint_Min
  RTCDiffTime : AIWAYS_Powertrain_BMS_lib/RTCCompare/RTCDiffTime
  Switch : Switch  Criteria=u2 ~= 0  Threshold=1  RndMeth=Zero
  TimeCompare : AIWAYS_Powertrain_BMS_lib/RTCCompare/TimeCompare
  LcRTC_IVICalSleepTime_s : Outport
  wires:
  GcADP_YearSet_Yr/1 -> Bus Creator/1
  GcADP_MonthSet_Mn/1 -> Bus Creator/2
  GcADP_DaySet_D/1 -> Bus Creator/3
  GcADP_HourSet_Hr/1 -> Bus Creator/4
  GcADP_MinSet_Min/1 -> Bus Creator/5
  GcADP_SecondSet_S/1 -> Bus Creator/6
  Data Store Read2/1 -> Bus Creator/7  "EcNVM_TimeYr_Yr"
  Data Store Read1/1 -> Bus Creator/8  "EcNVM_TimeMonth_M"
  Data Store Read3/1 -> Bus Creator/9  "EcNVM_TimeDay_D"
  Data Store Read4/1 -> Bus Creator/10  "EcNVM_TimeHr_Hr"
  Data Store Read6/1 -> Bus Creator/11  "EcNVM_TimeMint_Min"
  Data Store Read5/1 -> Bus Creator/12  "EcNVM_TimeSec_S"
  Bus Creator/1 -> Bus Selector2/1, Bus Selector3/1, Bus Selector/1, Bus Selector1/1
  Bus Selector/1 -> TimeCompare/1  "<GcADP_YearSet_Yr>"
  Bus Selector/2 -> TimeCompare/2  "<GcADP_MonthSet_Mn>"
  Bus Selector/3 -> TimeCompare/3  "<GcADP_DaySet_D>"
  Bus Selector/4 -> TimeCompare/4  "<GcADP_HourSet_Hr>"
  Bus Selector/5 -> TimeCompare/5  "<GcADP_MinSet_Min>"
  Bus Selector/6 -> TimeCompare/6  "<GcADP_SecondSet_S>"
  Bus Selector1/1 -> TimeCompare/7  "<EcNVM_TimeYr_Yr>"
  Bus Selector1/2 -> TimeCompare/8  "<EcNVM_TimeMonth_M>"
  Bus Selector1/3 -> TimeCompare/9  "<EcNVM_TimeDay_D>"
  Bus Selector1/4 -> TimeCompare/10  "<EcNVM_TimeHr_Hr>"
  Bus Selector1/5 -> TimeCompare/11  "<EcNVM_TimeMint_Min>"
  Bus Selector1/6 -> TimeCompare/12  "<EcNVM_TimeSec_S>"
  TimeCompare/1 -> Switch/2
  RTCDiffTime/1 -> Switch/1
  Bus Selector2/1 -> RTCDiffTime/1  "<GcADP_YearSet_Yr>"
  Bus Selector2/2 -> RTCDiffTime/2  "<GcADP_MonthSet_Mn>"
  Bus Selector2/3 -> RTCDiffTime/3  "<GcADP_DaySet_D>"
  Bus Selector2/4 -> RTCDiffTime/4  "<GcADP_HourSet_Hr>"
  Bus Selector2/5 -> RTCDiffTime/5  "<GcADP_MinSet_Min>"
  Bus Selector2/6 -> RTCDiffTime/6  "<GcADP_SecondSet_S>"
  Bus Selector3/1 -> RTCDiffTime/7  "<EcNVM_TimeYr_Yr>"
  Bus Selector3/2 -> RTCDiffTime/8  "<EcNVM_TimeMonth_M>"
  Bus Selector3/3 -> RTCDiffTime/9  "<EcNVM_TimeDay_D>"
  Bus Selector3/4 -> RTCDiffTime/10  "<EcNVM_TimeHr_Hr>"
  Bus Selector3/5 -> RTCDiffTime/11  "<EcNVM_TimeMint_Min>"
  Bus Selector3/6 -> RTCDiffTime/12  "<EcNVM_TimeSec_S>"
  Constant7/1 -> Switch/3
  Switch/1 -> LcRTC_IVICalSleepTime_s/1  "LcRTC_IVICalSleepTime_s"
